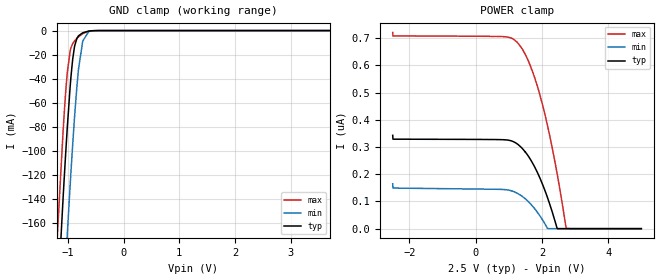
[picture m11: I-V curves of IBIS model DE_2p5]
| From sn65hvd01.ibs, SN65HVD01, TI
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|   Model
[Model]   DE_2p5
Model_type   Input
Vinl = 0.75
Vinh = 1.75
|   typ   min   max
C_comp   1pF   1pF   1pF
[Voltage Range]   2.5   2.25   2.75
[Temperature Range]   27   125   -40
[Power Clamp Reference]   2.5   2.25   2.75
[GND Clamp Reference]   -0   -0   -0
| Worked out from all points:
|   GND clamp passes 1 mA (typ) near -0.67 V on its own axis
[GND Clamp]
|   Voltage   I(typ)   I(min)   I(max)
-2.5V     -1.489A    -1.579A    -1.435A
-1.232V   -270.3mA   -366mA     -211mA
-1.083V   -139.6mA   -233mA     -83.95mA
-1.045V   -109.4mA   -201.1mA   -57.11mA
-1.008V   -81mA      -169.9mA   -35.07mA
-940mV    -37.75mA   -116.7mA   -14.16mA
-880mV    -14.05mA   -74.02mA   -8.816mA
-805mV    -4.333mA   -31.72mA   -5.166mA
-730mV    -1.837mA   -8.671mA   -2.539mA
-625mV    -447uA     -990.1uA   -553.1uA
-497.5mV  -41.81uA   -86.91uA   -34.69uA
4.992V    0A         0A         0A
[POWER Clamp]
|   Voltage   I(typ)   I(min)   I(max)
-2.5V     343.1nA    164.7nA    721.3nA
-2.493V   328.9nA    149.2nA    708.4nA
785mV     327.1nA    144.2nA    706nA
1.183V    316.9nA    134.4nA    692.4nA
1.385V    297.5nA    120.3nA    663.8nA
1.58V     267.8nA    100.3nA    618.6nA
1.768V    229.3nA    75.02nA    558.7nA
1.955V    180.7nA    43.57nA    482.9nA
2.165V    114.1nA    617.9pA    379nA
2.45V     3.007nA    0A         205.6nA
2.728V    0A         0A         1.319nA
4.992V    0A         0A         0A
